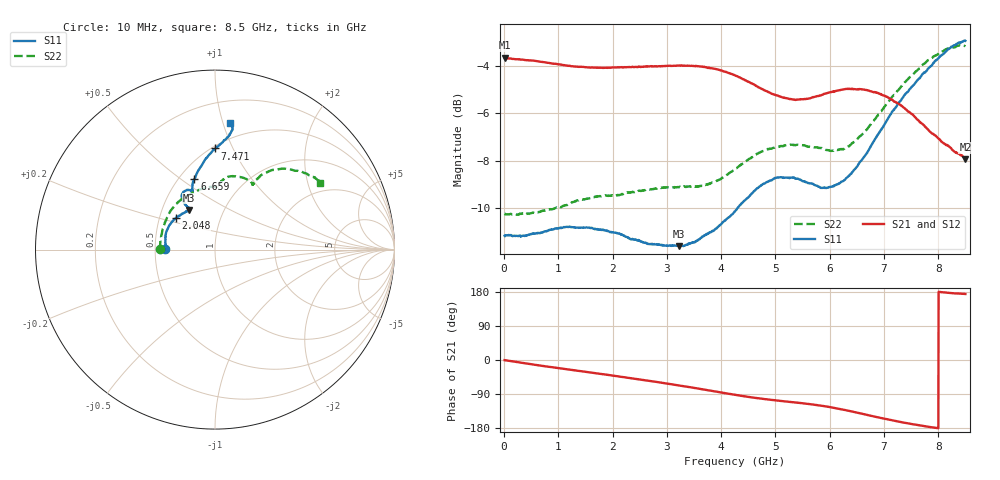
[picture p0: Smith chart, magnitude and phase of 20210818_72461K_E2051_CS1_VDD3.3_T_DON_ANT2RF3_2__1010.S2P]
!Agilent Technologies,E5071C,MY46417908,A.11.23
!Date: Wed Aug 18 14:29:51 2021
!Data & Calibration Information:
!Freq	S11:SOLT2(ON)	S21:SOLT2(ON)	S12:SOLT2(ON)	S22:SOLT2(ON)
!PortZ  Port1:50+j0  Port2:50+j0
!Above PortZ is port z conversion or system Z0 setting when saving the data.
!When reading, reference impedance value at option line is always used.
# Hz S dB R 50
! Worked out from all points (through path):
!   1601 points, 10 MHz to 8.5 GHz, reference 50 ohm
!   highest |S21| = -3.66 dB at 10 MHz (marker M1); lowest = -7.9 dB at 8.5 GHz (marker M2)
!   group delay of S21, straight-line fit = 61.7 ps
!   lowest |S11| = -11.6 dB at 3.22 GHz (marker M3), VSWR 1.71, Z = 34.3 + j16.3 ohm
!   |S11| at or under -10 dB: start of sweep to 4.297 GHz
!   |S22| runs from -10.3 to -3.1 dB; largest |S21 - S12| = 0.0038
!   S11 on the Smith chart (normalised r, x): 10 MHz: 0.57, +0.00; 2.048 GHz: 0.61, +0.23; 6.659 GHz: 0.60, +0.56; 7.471 GHz: 0.52, +0.86; 8.5 GHz: 0.37, +1.06
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1e7  -11.15 179.6  -3.66 -0.4  -3.66 -0.4  -10.22 179.8
5.671562e8  -11.07 171.3  -3.79 -12.5  -3.78 -12.5  -10.20 164.0
9.65125e8  -10.85 164.1  -3.92 -20.9  -3.91 -20.9  -9.97 151.7
1.426769e9  -10.81 154.7  -4.04 -29.9  -4.04 -29.9  -9.63 136.6
2.0476e9  -11.03 141.4  -4.06 -41.9  -4.07 -41.9  -9.46 117.3
2.843538e9  -11.53 126.1  -4.01 -58.6  -4.01 -58.7  -9.15 97.2
3.220281e9  -11.59 122.9  -3.99 -67.0  -3.99 -67.0  -9.11 91.9
3.692538e9  -11.13 122.0  -4.04 -78.2  -4.04 -78.3  -9.01 87.7
4.255e9  -10.13 123.3  -4.40 -91.8  -4.39 -91.8  -8.35 84.6
4.615825e9  -9.26 122.4  -4.80 -99.7  -4.80 -99.6  -7.77 80.6
5.003181e9  -8.73 118.9  -5.23 -106.5  -5.24 -106.5  -7.44 73.5
5.411762e9  -8.76 114.3  -5.42 -112.7  -5.43 -112.7  -7.32 65.4
5.671769e9  -8.96 112.1  -5.34 -117.1  -5.36 -117.2  -7.42 61.8
5.91055e9  -9.15 111.1  -5.17 -122.1  -5.20 -122.2  -7.52 60.3
6.191781e9  -8.93 111.0  -5.02 -129.3  -5.03 -129.5  -7.52 60.0
6.658731e9  -7.74 106.2  -5.01 -143.9  -5.00 -144.0  -6.74 59.1
7.088538e9  -6.16 97.4  -5.35 -157.4  -5.35 -157.5  -5.49 55.3
7.470588e9  -4.98 89.8  -5.95 -168.0  -5.95 -168.0  -4.49 49.0
7.714675e9  -4.34 85.5  -6.46 -174.0  -6.46 -174.1  -3.95 43.7
8.022438e9  -3.61 82.2  -7.09 179.6  -7.05 179.6  -3.45 37.8
8.351425e9  -3.06 82.4  -7.68 175.6  -7.64 175.6  -3.15 33.4
8.5e9  -2.94 83.1  -7.94 174.2  -7.86 174.2  -3.18 32.1
